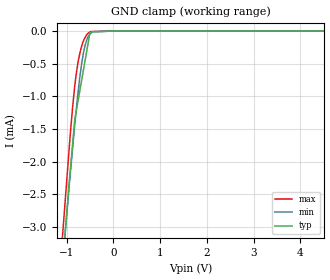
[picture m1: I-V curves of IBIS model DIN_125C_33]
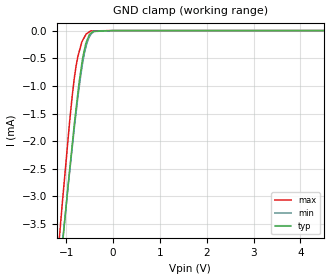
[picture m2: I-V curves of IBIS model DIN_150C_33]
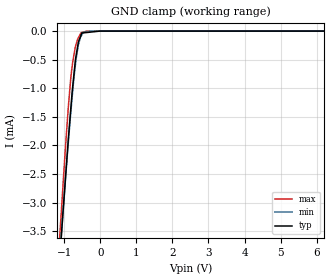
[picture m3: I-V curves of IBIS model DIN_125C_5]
|Texas Instruments Incorporated
|Programmable GAMMA-VOLTAGE GENERATOR
|   with Two High Slew Rate VCOMs
| Marketing part#   Digital Voltage Range   Package-type   #pins
|BUF18830AIRGFTR   2.0V to 5.5V   VQFN   38
[IBIS Ver]   4.0
[File name]   buf18830.ibs
[File Rev]   1.0
[Date]   05/19/2010
[Source]   Texas Instruments Incorporated.
   Analog-eLab, HPA
   12500 TI Blvd
   Dallas, TX -75243
   For Support e-mail: elab_ibis@list.ti.com
|   SIMDE - V2.0 201002 Build 453
[Notes]   Revision History:
   1.0: 05/19/2010
   - Initial version of the model
   - Initial Model generated from simulations in TISPICED
   - Model names with a trailing _33 contains the model for
   3.3V (3.0V and 3.6V).
   _ Model names with trailing _5 contains
   the model for 5V (4.5V and 5.5V) operation.
   - Model not matched to measurements
   - C_comp although listed in numerical order of value are
   obtained from varying PVT conditions. For PVT conditions
   for each specific value refer the buffer description under
   respective [Model]. IBIS model user is responsible for using
   appropriate C_comp to simulate for Signal Integrity.
   - Combined Pulldown non-monotonic warnings for SDA_150C_5,
   SDA_125C_5, SDA_150C_33, and SDA_125C_33 typical, minimum,
   and maximum errors are minimal and accepted.
[Disclaimer]
 This product is designed as an aid for customers of Texas Instruments.
 No warranties, either expressed or implied, with respect to this third
 party software (if any) or with respect to its fitness for any
 particular purpose is claimed by Texas Instruments or the author. The
 software (if any) is provided solely on an "as is" basis. The entire
 risk as to its quality and performance is with the customer
[Copyright] (C) Copyright 2011 Texas Instruments Incorporated.
   All rights reserved.
|   BUF18830
[Component]   buf18830rge
[Manufacturer] TI
[Package]   | 38 VQFN - RGF package
| variable   typ   min   max
R_pkg   0.03330   0.02235   0.05888
L_pkg   1.35521nH 0.97700nH 1.77220nH
C_pkg   0.30234pF 0.22913pF 0.34486pF
|-------------------------PIN------------------------------------------------
[Pin] signal_name  model_name  R_pin  L_pin C_pin
1   AVDD-VCOM   POWER   0.03367  1.70924nH  0.29829pF
2   VCOM-OUT2   TERM   0.03024  1.49535nH  0.31090pF
3   VCOM-FEEDBACK2  TERM   0.05376  1.60996nH  0.25594pF
4   DVDD   POWER   0.05247  1.56701nH  0.24169pF
5   SCL   DIN   0.04888  1.44780nH  0.23480pF
6   SDA   SDA   0.04676  1.37769nH  0.22922pF
7   A0   DIN   0.04610  1.35589nH  0.22913pF
8   DVSS   GND   0.04749  1.40170nH  0.23774pF
9   GND-VCOM   GND   0.02541  1.17477nH  0.29017pF
10  VCOM-FEEDBACK1  TERM   0.05453  1.63566nH  0.26410pF
11  VCOM-OUT1   TERM   0.03070  1.52678nH  0.31650pF
12  AVDD-VCOM   POWER   0.03376  1.71990nH  0.30217pF
13  AVDD   POWER   0.03168  1.52009nH  0.33119pF
14  OUT0   TERM   0.02968  1.40421nH  0.33766pF
15  OUT1   TERM   0.02848  1.32575nH  0.32908pF
16  OUT2   TERM   0.02808  1.29797nH  0.32557pF
17  OUT3   TERM   0.02850  1.32298nH  0.32904pF
18  OUT4   TERM   0.02971  1.39880nH  0.33824pF
19  OUT5   TERM   0.03174  1.52081nH  0.33178pF
20  GND   GND   0.02249  1.71649nH  0.34373pF
21  GND   GND   0.06009  1.81339nH  0.28456pF
22  AVDD   POWER   0.01909  1.21161nH  0.35762pF
23  OUT6   TERM   0.02710  1.28773nH  0.31272pF
24  OUT7   TERM   0.02468  1.12862nH  0.30384pF
25  OUT8   TERM   0.02303  1.02126nH  0.28946pF
26  OUT9   TERM   0.02235  0.97700nH  0.28364pF
27  OUT10   TERM   0.02276  1.00159nH  0.28719pF
28  OUT11   TERM   0.02419  1.09688nH  0.29959pF
29  GND   GND   0.02644  1.24442nH  0.30752pF
30  TSENSE   TERM   0.05888  1.77220nH  0.26970pF
31  AVDD   POWER   0.03354  1.79663nH  0.29784pF
32  OUT12   TERM   0.03070  1.45267nH  0.31941pF
33  OUT13   TERM   0.02901  1.35853nH  0.33215pF
34  OUT14   TERM   0.02819  1.30516nH  0.32644pF
35  OUT15   TERM   0.02818  1.30407nH  0.32644pF
36  OUT16   TERM   0.02899  1.35527nH  0.33333pF
37  OUT17   TERM   0.03054  1.45487nH  0.34486pF
38  GND   GND   0.03285  1.59748nH  0.33709pF
|   Model Selectors
[Model Selector]  DIN
DIN_125C_33   3.3V digital input
DIN_150C_33   3.3V digital input
DIN_125C_5   5V digital input
DIN_150C_5   5V digital input
|NOTES   Model DIN split into four Models DIN_125C_33, DIN_150C_33,
|   DIN_125C_5 and DIN_150C_5 to accomodate vast voltage range of
|   2.0V - 5.5V and junction temperatures up to 150C.
|   DIN_125C_33 operates in voltage range of 3.0 - 3.3 - 3.6 with
|   junction temperature tests at -40, 67, and 125C.
|   Power dissipated equals 1.13A.
|   DIN_150C_33 operates in voltage range of 3.0 - 3.3 - 3.6 with
|   junction temperature tests at -40, 92, and 150C.
|   Power dissipated equals 1.8A.
|   DIN_125C_5 operates in voltage range of 4.5 - 5.0 - 5.5 with
|   junction temperature tests at -40, 67, and 125C.
|   Power dissipated equals 1.13A.
|   DIN_150C_5 operates in voltage range of 4.5 - 5.0 - 5.5 with
|   junction temperature tests at -40, 92, and 150C.
|   Power dissipated equals 1.8A.
|   The max pin frequency for Model DIN is 3.4MHz.Also the
|   voltage range and frequency is referenced with datasheet.
[Model Selector]  SDA
SDA_125C_33  3.3V digital output
SDA_150C_33  3.3V digital output
SDA_125C_5   5V digital output
SDA_150C_5   5V digital output
|NOTES   Model SDA split into four Models SDA_125C_33, SDA_150C_33,
|   SDA_125C_5 and SDA_150C_5 to accomodate vast voltage range of
|   2.0V - 5.5V and junction temperatures up to 150C.
|   SDA_125C_33 operates in voltage range of 3.0 - 3.3 - 3.6 with
|   junction temperature tests at -40, 67, and 125C.
|   Power dissipated equals 1.13A.
|   SDA_150C_33 operates in voltage range of 3.0 - 3.3 - 3.6 with
|   junction temperature tests at -40, 92, and 150C.
|   Power dissipated equals 1.8A.
|   SDA_125C_5 operates in voltage range of 4.5 - 5.0 - 5.5 with
|   junction temperature tests at -40, 67, and 125C.
|   Power dissipated equals 1.13A.
|   SDA_150C_5 operates in voltage range of 4.5 - 5.0 - 5.5 with
|   junction temperature tests at -40, 92, and 150C.
|   Power dissipated equals 1.8A.
|   The max pin frequency for Model SDA is 3.4MHz.Also the
|   voltage range and frequency is referenced with datasheet.
[Model Selector]  TERM
TERM_125C_33  3.3V digital output
TERM_150C_33  3.3V digital output
TERM_125C_5   5V digital output
TERM_150C_5   5V digital output
|   TERM Models
[Model] TERM_125C_33
Model_type Terminator
C_comp   1e-200   1e-200   1e-200
| variable   typ   min   max
[Voltage Range]   3.3   3   3.6
|Operating Temperature   27   95   -40
[Temperature Range]   67   125   -40
[Model] TERM_150C_33
Model_type Terminator
C_comp   1e-200   1e-200   1e-200
| variable   typ   min   max
[Voltage Range]   3.3   3   3.6
|Operating Temperature   27   95   -40
[Temperature Range]   92   150   -40
[Model] TERM_125C_5
Model_type Terminator
C_comp   1e-200   1e-200   1e-200
| variable   typ   min   max
[Voltage Range]   5   4.5   5.5
|Operating Temperature   27   95   -40
[Temperature Range]   67   125   -40
[Model] TERM_150C_5
Model_type Terminator
C_comp   1e-200   1e-200   1e-200
| variable   typ   min   max
[Voltage Range]   5   4.5   5.5
|Operating Temperature   27   95   -40
[Temperature Range]   92   150   -40
| Models and submodels in the file (12): DIN_125C_33 (Input), DIN_150C_33 (Input), DIN_125C_5 (Input), DIN_150C_5 (Input), SDA_125C_33 (I/O_open_drain), SDA_150C_33 (I/O_open_drain), SDA_125C_5 (I/O_open_drain), SDA_150C_5 (I/O_open_drain), TERM_125C_33 (Terminator), TERM_150C_33 (Terminator), TERM_125C_5 (Terminator), TERM_150C_5 (Terminator)
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|NOTES   Model TERM split into four Models TERM_125C_33, TERM_150C_33,
|   TERM_125C_5 and TERM_150C_5 to accomodate vast voltage range of
|   2.0V - 5.5V and junction temperatures up to 150C.
|   TERM_125C_33 operates in voltage range of 3.0 - 3.3 - 3.6 with
|   junction temperature tests at -40, 67, and 125C.
|   Power dissipated equals 1.13A.
|   TERM_150C_33 operates in voltage range of 3.0 - 3.3 - 3.6 with
|   junction temperature tests at -40, 92, and 150C.
|   Power dissipated equals 1.8A.
|   TERM_125C_5 operates in voltage range of 4.5 - 5.0 - 5.5 with
|   junction temperature tests at -40, 67, and 125C.
|   Power dissipated equals 1.13A.
|   TERM_150C_5 operates in voltage range of 4.5 - 5.0 - 5.5 with
|   junction temperature tests at -40, 92, and 150C.
|   Power dissipated equals 1.8A.
|   DIN_33 Models
[Model] DIN_125C_33
|Signals
Model_type Input
Vinl = 0.99
Vinh = 2.31
|   typ   min   max
|   (nom PVT)   (Fast PVT)   (slow PVT)
C_comp   5.49642E-13   5.37132E-13   5.70282E-13
| Where   nom PVT is  Nominal Process, 3.3V, 67C
|   Fast PVT is Strong Process, 3.6V, -40C
|   Slow PVT is Weak Process, 3.0V, 125C
[Model Spec]   |3.3V model
Vinl   0.99   0.9   1.08
Vinh   2.31   2.1   2.52
|Vinl = 0.3 X DVDD
|Vinh = 0.7 X DVDD
[Voltage Range]   3.3   3   3.6
|Operating Temperature   27   85   -40
[Temperature Range]   67   125   -40
[Power Clamp Reference]   3.3   3   3.6
[GND Clamp Reference]   0   0   0
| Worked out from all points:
|   GND clamp passes 1 mA (typ) near -0.74 V on its own axis
[GND Clamp]
|   Voltage   I(typ)   I(min)   I(max)
-3.3V     -25.16mA   -23.94mA   -26.88mA
-1.084V   -3.566mA   -3.546mA   -3.116mA
-940.6mV  -2.302mA   -2.341mA   -1.766mA
-869.4mV  -1.721mA   -1.783mA   -1.156mA
-825mV    -1.36mA    -1.436mA   -839.7uA
-791.3mV  -1.221mA   -1.196mA   -645.6uA
-718.3mV  -921.6uA   -717.2uA   -348.6uA
-638.3mV  -592.9uA   -331.6uA   -151.9uA
-553.4mV  -244uA     -107.8uA   -44uA
-499.8mV  -24.13uA   -42.4uA    -14.3uA
-476.5mV  -14.77uA   -29.91uA   -5.98uA
6.59V     0A         0A         0A
[POWER Clamp]
|   SCR cell for ESD function. Effects occurr above VDD x 2
|   Voltage   I(typ)   I(min)   I(max)
-3.3V     0A         0A         0A
0V        0A         0A         0A
6.6V      0A         0A         0A
[Model] DIN_150C_33
|Signals
Model_type Input
Vinl = 0.99
Vinh = 2.31
|   typ   min   max
|   (nom PVT)   (Fast PVT)   (slow PVT)
C_comp   5.49642E-13   5.37132E-13   5.88954E-13
| Where   nom PVT is  Nominal Process, 3.3V, 92C
|   Fast PVT is Strong Process, 3.6V, -40C
|   Slow PVT is Weak Process, 3.0V, 150C
[Model Spec]   |3.3V model
Vinl   0.99   0.9   1.08
Vinh   2.31   2.1   2.52
|Vinl = 0.3 X DVDD
|Vinh = 0.7 X DVDD
[Voltage Range]   3.3   3   3.6
|Operating Temperature   27   85   -40
[Temperature Range]   92   150   -40
[Power Clamp Reference]   3.3   3   3.6
[GND Clamp Reference]   0   0   0
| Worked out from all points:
|   GND clamp passes 1 mA (typ) near -0.73 V on its own axis
[GND Clamp]
|   Voltage   I(typ)   I(min)   I(max)
-3.3V     -25.2mA    -24.01mA   -26.88mA
-1.3V     -5.874mA   -5.749mA   -5.288mA
-1.125V   -4.26mA    -4.2mA     -3.522mA
-1.086V   -3.912mA   -3.873mA   -3.138mA
-920.5mV  -2.46mA    -2.496mA   -1.582mA
-869.4mV  -2.035mA   -2.09mA    -1.156mA
-791.3mV  -1.419mA   -1.49mA    -645.6uA
-649.1mV  -490.6uA   -579.8uA   -176.5uA
-580.4mV  -224.8uA   -296.8uA   -69.47uA
-476.5mV  -47.43uA   -71.64uA   -5.98uA
-5.69mV   -10.56nA   0A         0A
6.59V     0A         0A         0A
[POWER Clamp]
|   SCR cell for ESD function. Effects occurr above VDD x 2
|   Voltage   I(typ)   I(min)   I(max)
-3.3V     0A         0A         0A
0V        0A         0A         0A
6.6V      0A         0A         0A
|   INPUT 5V Models
[Model]   DIN_125C_5   |Rload to VDD = 1k ohms
Model_type   Input
|Signals
Vinl = 1.5
Vinh = 3.5
|   typ   min   max
|   (Fast PVT)   (Nom PVT)   (slow PVT)
C_comp   5.59861E-13   5.37132E-13   5.80873E-13
| Where   Nom PVT is  Nominal Process, 5.0V, 67C
|   Fast PVT is Strong Process, 5.5V, -40C
|   Slow PVT is Weak Process, 4.5V, 125C
[Model Spec]   |5V model
Vinl   1.5   1.35   1.65
Vinh   3.5   3.15   3.85
|Vinl = 0.3 X DVDD
|Vinh = 0.7 X DVDD
[Voltage Range]   5   4.5   5.5
|Operating Temperature   27   85   -40
[Temperature Range]   67   125   -40
[Power Clamp Reference]   5   4.5   5.5
[GND Clamp Reference]   0   0   0
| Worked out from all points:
|   GND clamp passes 1 mA (typ) near -0.77 V on its own axis
[GND Clamp]
|   Voltage   I(typ)   I(min)   I(max)
-5V       -42.09mA   -39.94mA   -45.76mA
-1.233V   -4.94mA    -4.846mA   -4.602mA
-1.052V   -3.277mA   -3.295mA   -2.825mA
-979.4mV  -2.649mA   -2.674mA   -2.115mA
-891.4mV  -1.889mA   -1.953mA   -1.334mA
-803.4mV  -1.208mA   -1.287mA   -710.1uA
-690mV    -484.4uA   -566.4uA   -264.3uA
-611.4mV  -190.3uA   -241.5uA   -115.1uA
-529.3mV  -56.85uA   -82.46uA   -24.67uA
-474mV    -30.96uA   -23.88uA   -16.13uA
-279.2mV  -18.11uA   -133.9nA   -97.7nA
9.985V    0A         0A         0A
|DVDD = 5V
[POWER Clamp]
|   SCR cell for ESD function. Effects occurr above VDD x 2
|   Voltage   I(typ)   I(min)   I(max)
-5V       0A         0A         0A
0V        0A         0A         0A
10V       0A         0A         0A
